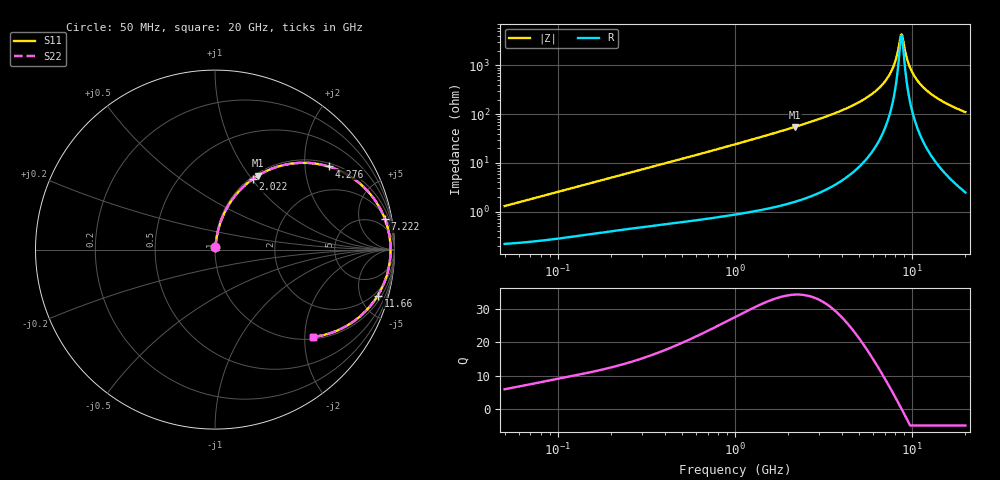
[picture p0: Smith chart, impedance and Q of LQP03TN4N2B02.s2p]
!Murata Part Number: LQP03TN4N2B02
!These Parameters are Measured in Series Mode Connection
!  o--[Z]--o
!Port1  Port2
!  o-------o
!Freq. Start=50[MHz] Stop=20[GHz], 401[Steps]
# Hz S RI R 50
!Freq.(Hz) S11(Real) S11(Imag) S21(Real) S21(Imag) S12(Real) S12(Imag) S22(Real) S22(Imag)
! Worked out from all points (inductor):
!   401 points, 50 MHz to 20 GHz, reference 50 ohm
!   read as one part in series: L = 4.08 nH near 51.52 MHz
!   highest Q = 34.4 at 2.179 GHz (marker M1), where L = 4.01 nH
!   self-resonance near 8.645 GHz
!   S11 on the Smith chart (normalised r, x): 50 MHz: 1.00, +0.03; 2.022 GHz: 1.03, +1.01; 4.276 GHz: 1.10, +2.65; 7.222 GHz: 2, +11; 11.66 GHz: 1.51, -6.91; 20 GHz: 1.05, -2.21
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5e7  0.00235 0.0128  0.9977 -0.0128  0.9977 -0.0128  0.00235 0.0128
1.364002e8  0.00442 0.034  0.9956 -0.034  0.9956 -0.034  0.00442 0.034
3.721004e8  0.0133 0.0888  0.9867 -0.0888  0.9867 -0.0888  0.0133 0.0888
1e9  0.0622 0.2241  0.9378 -0.2241  0.9378 -0.2241  0.0622 0.2241
2.021818e9  0.2099 0.3929  0.7901 -0.3929  0.7901 -0.3929  0.2099 0.3929
2.179053e9  0.2379 0.4115  0.7621 -0.4115  0.7621 -0.4115  0.2379 0.4115
2.728004e9  0.3416 0.4597  0.6584 -0.4597  0.6584 -0.4597  0.3416 0.4597
4.275624e9  0.6324 0.4633  0.3676 -0.4633  0.3676 -0.4633  0.6324 0.4633
5.856089e9  0.848 0.3291  0.152 -0.3291  0.152 -0.3291  0.848 0.3291
6.601595e9  0.9113 0.2441  0.0887 -0.2441  0.0887 -0.2441  0.9113 0.2441
7.222371e9  0.9466 0.1705  0.0534 -0.1705  0.0534 -0.1705  0.9466 0.1705
7.442007e9  0.9556 0.1445  0.0444 -0.1445  0.0444 -0.1445  0.9556 0.1445
8.020766e9  0.9718 0.0771  0.0282 -0.0771  0.0282 -0.0771  0.9718 0.0771
8.516016e9  0.9777 0.0217  0.0223 -0.0217  0.0223 -0.0217  0.9777 0.0217
8.774992e9  0.9783 -0.00625  0.0217 0.00625  0.0217 0.00625  0.9783 -0.00625
8.907419e9  0.9779 -0.0202  0.0221 0.0202  0.0221 0.0202  0.9779 -0.0202
9.457416e9  0.9727 -0.0758  0.0273 0.0758  0.0273 0.0758  0.9727 -0.0758
9.892087e9  0.9646 -0.1167  0.0354 0.1167  0.0354 0.1167  0.9646 -0.1167
1.066139e10  0.9436 -0.1826  0.0564 0.1826  0.0564 0.1826  0.9436 -0.1826
1.166392e10  0.9071 -0.2558  0.0929 0.2558  0.0929 0.2558  0.9071 -0.2558
1.460232e10  0.7744 -0.3987  0.2256 0.3987  0.2256 0.3987  0.7744 -0.3987
2e10  0.548 -0.4865  0.452 0.4865  0.452 0.4865  0.548 -0.4865
